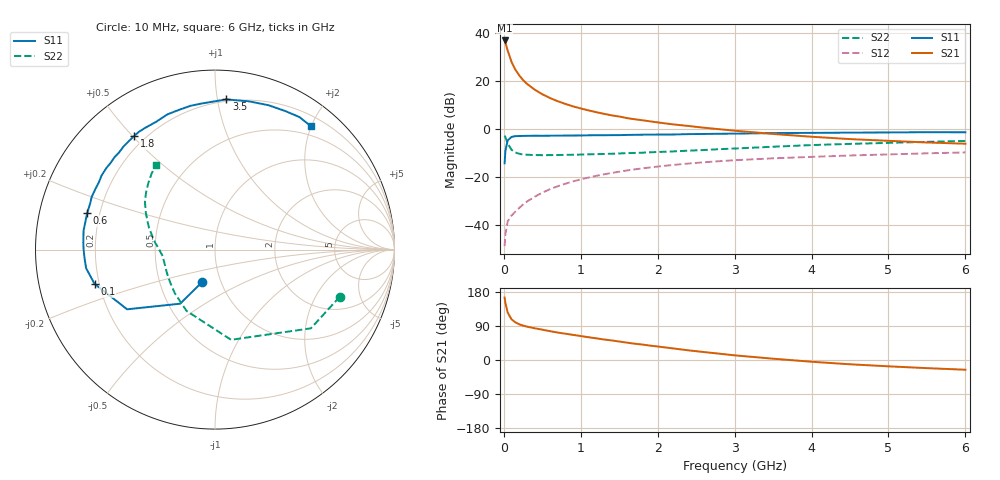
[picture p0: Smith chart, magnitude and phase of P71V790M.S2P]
! SIEMENS Small Signal Semiconductors
! BFP196
! Si NPN RF Bipolar Junction Transistor in SOT143
! VCE = 1.75 V  IC = 90 mA
! Common Emitter S-Parameters:  May  1996
# GHz  S  MA  R  50
!  f  S11  S21  S12  S22
! GHz  MAG  ANG  MAG  ANG  MAG  ANG  MAG  ANG
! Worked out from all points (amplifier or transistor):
!   36 points, 10 MHz to 6 GHz, reference 50 ohm
!   highest |S21| = 37.1 dB at 10 MHz (marker M1)
!   |S21| within 3 dB of that: start of sweep to 39.07 MHz
!   unconditionally stable (mu >= 1): 264.8 MHz to 5.352 GHz; 5.619 GHz to end of sweep
!   at 250 MHz: K = 0.99, MSG = 25.9 dB, |S12| = -31.3 dB
!   at 1.4 GHz: K = 1.11, MAG = 10.0 dB, |S12| = -18.1 dB
!   at 6 GHz: K = 1.02, MAG = 1.0 dB, |S12| = -9.6 dB
!   S11 on the Smith chart (normalised r, x): 10 MHz: 0.81, -0.31; 100 MHz: 0.18, -0.14; 600 MHz: 0.15, +0.14; 1.8 GHz: 0.16, +0.50; 3.5 GHz: 0.19, +1.06; 6 GHz: 0.35, +2.00
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0.01  0.1969 -111.9  71.35 164.8  0.0037 70.9  0.7433 -20.7
0.02  0.3585 -122.8  64.72 150.6  0.0065 64.0  0.6911 -39.4
0.05  0.5918 -145.8  43.82 125.1  0.0121 53.0  0.5105 -79.9
0.1  0.6977 -164.1  25.49 107.3  0.0161 51.1  0.3765 -114.9
0.15  0.7255 -171.8  17.56 99.3  0.0194 55.4  0.3309 -132.5
0.2  0.7289 -176.6  13.36 94.2  0.0231 59.3  0.3109 -142.9
0.25  0.7323 179.6  10.67 90.8  0.0273 60.9  0.3016 -150.3
0.3  0.7348 176.9  8.931 88.1  0.0314 63.8  0.297 -154.8
0.4  0.74 171.7  6.759 83.8  0.0396 65.7  0.2924 -161.4
0.5  0.7384 168.4  5.407 80.0  0.0481 66.6  0.2912 -165.6
0.6  0.7407 164.0  4.506 76.1  0.057 66.9  0.2918 -168.5
0.7  0.7411 160.1  3.874 72.4  0.0654 66.3  0.293 -170.7
0.8  0.747 156.9  3.398 69.4  0.074 65.3  0.2952 -172.5
1.1  0.7547 146.9  2.494 60.1  0.0994 62.2  0.3025 -176.8
1.4  0.7606 137.3  1.966 51.7  0.1238 57.8  0.3117 179.7
1.8  0.7767 125.5  1.553 40.8  0.1544 51.5  0.3273 175.2
2.2  0.784 114.7  1.275 30.5  0.182 45.3  0.3484 170.1
2.8  0.8126 99.7  1.011 16.7  0.2179 36.0  0.3878 161.6
3.5  0.8394 85.7  0.805 3.4  0.2501 25.6  0.4362 152.0
4.5  0.8578 69.7  0.629 -11.3  0.2863 13.4  0.5001 140.1
5.5  0.8756 57.5  0.535 -21.5  0.3179 2.5  0.551 129.9
6  0.8709 52.1  0.504 -25.7  0.332 -3.2  0.5753 125.0
